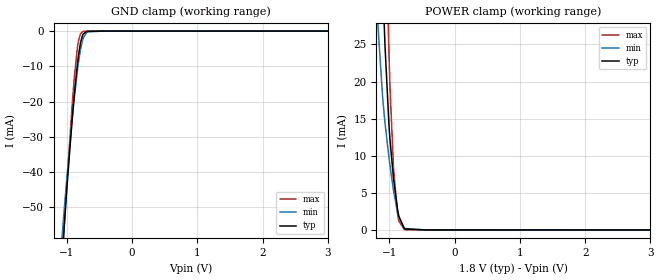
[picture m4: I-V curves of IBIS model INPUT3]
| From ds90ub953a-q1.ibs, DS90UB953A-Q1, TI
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|   INPUT3 Model
[Model]   INPUT3
Model_type   Input
Vinl = 0.63
Vinh = 1.17
|   typ   min   max
C_comp   0.1854pF   0.14pF   0.2275pF
| Where Nom  PVT is Nominal Process, 1.8V, 27C
|   Fast PVT is Strong Process,  1.89V, -40C
|   Slow PVT is Weak Process,   1.71V, 105C
[Model spec]
|subparameter
Vinl   0.63   0.5985   0.6615
Vinh   1.17   1.1115   1.2285
[Voltage Range]   1.8   1.71   1.89
|Junction Temperature
[Temperature Range]   27   105   -40
[Power Clamp Reference]   1.8   1.71   1.89
[GND Clamp Reference]   0   0   0
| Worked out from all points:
|   GND clamp passes 1 mA (typ) near -0.75 V on its own axis
|   POWER clamp passes 1 mA (typ) near -0.81 V on its own axis
[GND Clamp]
|   Voltage   I(typ)   I(min)   I(max)
-1.8V     -284.8mA   -258.7mA   -304.1mA
-1.157V   -88.28mA   -78.94mA   -91.88mA
-1.06V    -60.69mA   -55.12mA   -61.4mA
-1.017V   -49.03mA   -45.3mA    -48.33mA
-919.8mV  -25.17mA   -25.2mA    -21.19mA
-882mV    -17.19mA   -18.26mA   -12.34mA
-838.8mV  -9.383mA   -11.23mA   -4.644mA
-822.6mV  -6.953mA   -8.932mA   -2.754mA
-763.2mV  -1.4mA     -2.823mA   -210uA
-676.8mV  -51.64uA   -230.9uA   -4.149uA
-444.6mV  -450.8nA   -488.9nA   -548nA
3.6V      0A         0A         0A
[POWER Clamp]
|   Voltage   I(typ)   I(min)   I(max)
-1.8V     329.6mA    247.7mA    397.8mA
-1.179V   58.29mA    28.05mA    92.07mA
-1.103V   34mA       17.88mA    59.14mA
-1.076V   27.04mA    15.27mA    48.23mA
-1.066V   24.56mA    14.32mA    44.04mA
-1.006V   14.15mA    9.74mA     23.68mA
-990mV    12.11mA    8.63mA     19.17mA
-936mV    6.875mA    5.294mA    8.276mA
-876.6mV  2.883mA    2.414mA    2.297mA
-855mV    1.854mA    1.647mA    1.184mA
-768.6mV  134.4uA    202.8uA    32.78uA
3.6V      0A         0A         0A
